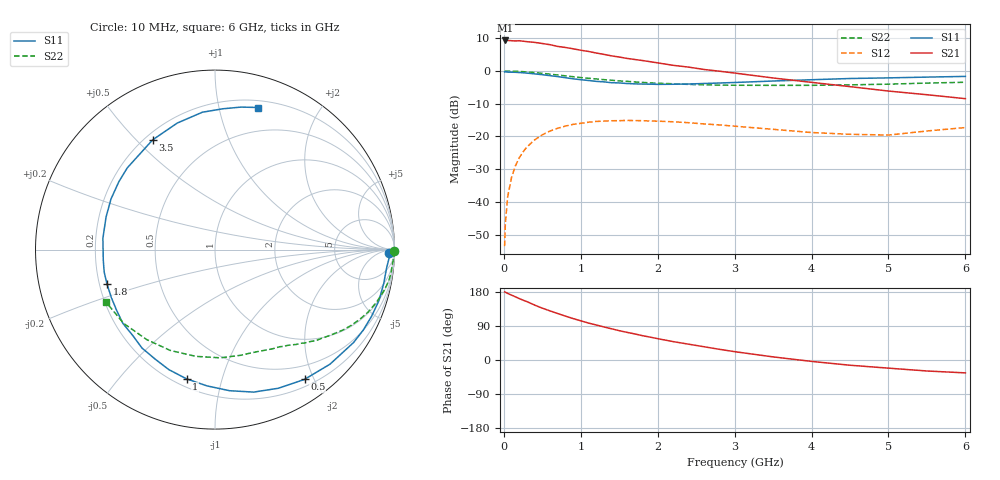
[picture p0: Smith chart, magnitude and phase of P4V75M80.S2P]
! SIEMENS Small Signal Semiconductors
! BFP182
! Si NPN RF Bipolar Junction Transistor in SOT143
! VCE = 0.75 V  IC = 0.8 mA
! Common Emitter S-Parameters:  March  1996
# GHz  S  MA  R  50
!  f  S11  S21  S12  S22
! GHz  MAG  ANG  MAG  ANG  MAG  ANG  MAG  ANG
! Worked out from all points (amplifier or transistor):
!   36 points, 10 MHz to 6 GHz, reference 50 ohm
!   highest |S21| = 9.3 dB at 20 MHz (marker M1)
!   |S21| within 3 dB of that: start of sweep to 1.003 GHz
!   unconditionally stable (mu >= 1): 2.59 GHz to end of sweep
!   at 250 MHz: K = 0.10, MSG = 16.9 dB, |S12| = -24.7 dB
!   at 1.4 GHz: K = 0.55, MSG = 9.9 dB, |S12| = -15.2 dB
!   at 6 GHz: K = 1.35, MAG = 0.9 dB, |S12| = -17.3 dB
!   S11 on the Smith chart (normalised r, x): 10 MHz: 45, -26; 500 MHz: 0.30, -1.87; 1 GHz: 0.25, -0.77; 1.8 GHz: 0.23, -0.15; 3.5 GHz: 0.23, +0.56; 6 GHz: 0.26, +1.32
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0.01  0.9672 -1.1  2.925 179.6  0.0021 84.6  0.9981 -0.5
0.02  0.9728 -2.3  2.933 179.0  0.0047 89.9  0.9958 -0.9
0.05  0.962 -5.9  2.933 175.6  0.012 86.7  0.9974 -2.3
0.1  0.9588 -11.4  2.907 171.2  0.0236 81.8  0.9916 -4.7
0.15  0.9567 -17.2  2.881 166.8  0.0354 78.8  0.9895 -7.1
0.2  0.9484 -23.0  2.902 162.2  0.0471 75.6  0.986 -9.3
0.3  0.9297 -33.8  2.811 154.1  0.0689 68.4  0.9674 -13.9
0.4  0.9045 -44.9  2.741 145.0  0.0885 61.8  0.9468 -18.0
0.5  0.8784 -55.4  2.634 136.8  0.1058 55.0  0.922 -22.1
0.6  0.8495 -65.4  2.527 129.6  0.1209 49.0  0.8955 -25.7
0.8  0.7904 -84.1  2.293 115.8  0.1439 38.4  0.8443 -31.9
1  0.7374 -102.4  2.079 103.4  0.1586 29.0  0.7947 -37.2
1.1  0.7165 -111.0  1.993 97.5  0.165 24.9  0.7743 -39.6
1.5  0.6576 -141.3  1.636 77.4  0.174 11.0  0.706 -47.7
1.8  0.6317 -162.3  1.448 64.3  0.174 3.6  0.6699 -52.8
2.2  0.6277 174.3  1.223 48.6  0.1675 -5.2  0.6386 -60.0
2.8  0.6557 144.8  0.994 28.3  0.15 -13.4  0.6088 -71.5
3.5  0.7033 119.6  0.783 8.2  0.1285 -17.4  0.6037 -87.2
4.5  0.7685 95.3  0.577 -13.8  0.1078 -10.3  0.6147 -113.9
5  0.7856 86.9  0.494 -21.5  0.1049 -1.0  0.6295 -127.3
5.5  0.8073 79.6  0.434 -29.0  0.1211 3.5  0.6543 -141.1
6  0.8274 73.1  0.378 -34.0  0.1366 4.6  0.6734 -154.1
